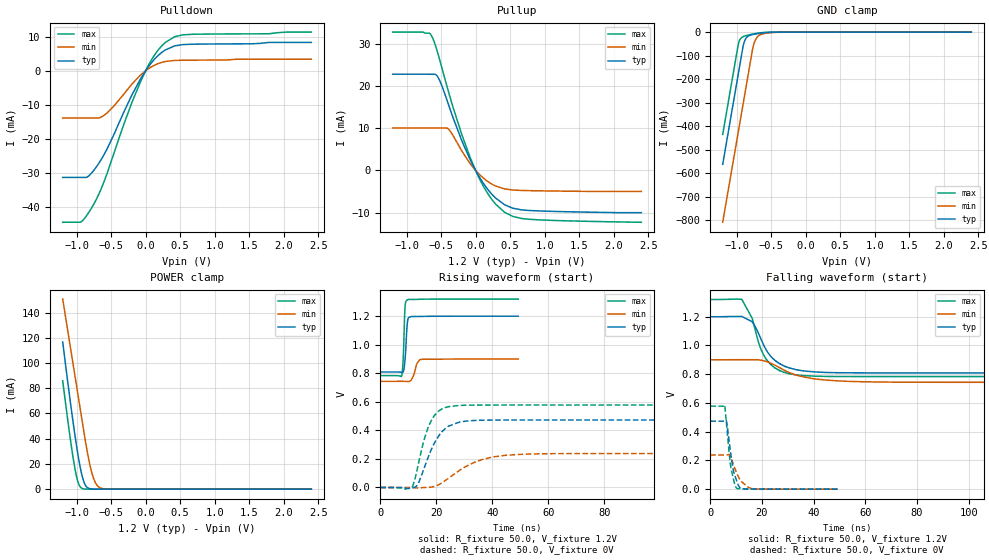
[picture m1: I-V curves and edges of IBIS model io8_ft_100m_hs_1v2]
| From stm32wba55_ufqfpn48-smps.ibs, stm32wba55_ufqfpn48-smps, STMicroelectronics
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[Model]   io8_ft_100m_hs_1v2
Model_type I/O
Polarity   Non-Inverting
Enable   Active-Low
| CAP_THRESHOLD on pad IOFT is "UDTCAPC" :
| Rising=30.0% of vddiom   Falling=70.0% of vddiom
| C_comp min and max val. don't necessarily correlate with the min and max pvt
| but are the smallest and greatest pad capacitance found.
| var   typ   min   max
C_comp   1.75103pF  1.57484pF  1.87847pF
|C_comp_pullup   1.05650pF  962.72500fF  1.08780pF
|C_comp_pulldown   694.52500fF  612.11500fF  790.67000fF
Vinl = 450.0mV
Vinh = 660.0mV
Vmeas = 600.0mV   | Reference voltage for timing measurements
Cref  = 50.0pF   | Timing specification test load capacitance value
Rref  = 1.0MOhm   | Timing specification test load resistance value
Vref  = 660.0mV   | Timing specification test load voltage
[Model Spec]
| TIME_THRESHOLD on pin ZIV11 is "CMOS" :
| Rising=50.0% of vdd   Falling=50.0% of vdd
Vinl 441.50000mV 347.50000mV 471.50000mV
Vinh 755.50000mV 552.50000mV 842.50000mV
| variable   typ   min   max
[Temperature Range] 25.0 140.0 -40.0
| variable   typ   min   max
[Voltage Range] 1.2V 900.0mV 1.32V
| variable   typ   min   max
[POWER Clamp Reference] 1.2V 900.0mV 1.32V
| variable   typ   min   max
[GND Clamp Reference] 0V 0V 0V
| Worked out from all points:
|   slope of the pulldown table from 0 to 0.18 V, typ, clamps not added: 40.6 ohm
|   slope of the pullup table from 0 to 0.18 V, typ, clamps not added: 39.4 ohm
|   GND clamp passes 1 mA (typ) near -0.51 V on its own axis
|   POWER clamp passes 1 mA (typ) near -0.83 V on its own axis
|   rising waveform, R_fixture 50.0, V_fixture 1.2V: 20-80 % time 738ps typ, 1.44ns min, 563ps max; typ from 0.809 V to 1.2 V
|   falling waveform, R_fixture 50.0, V_fixture 1.2V: 20-80 % time 8.08ns typ, 13.6ns min, 6.71ns max; typ from 1.2 V to 0.809 V
|   rising waveform, R_fixture 50.0, V_fixture 0V: 20-80 % time 6.62ns typ, 12.4ns min, 5ns max; typ from 0 V to 0.473 V
|   falling waveform, R_fixture 50.0, V_fixture 0V: 20-80 % time 2.5ns typ, 3.86ns min, 2.13ns max; typ from 0.473 V to 0 V
[POWER Clamp]
-1.2V     116.7mA    150.7mA    85.92mA
-1.06V    57.23mA    102.6mA    28.68mA
-1.02V    41.75mA    88.91mA    15.5mA
-980mV    27.6mA     75.18mA    5.935mA
-920mV    10.75mA    54.6mA     597.6uA
-870mV    3.065mA    37.68mA    60.82uA
-820mV    594.6uA    22.85mA    5.912uA
-770mV    99.71uA    11.47mA    572nA
-730mV    23.34uA    5.552mA    88.29nA
-680mV    3.779uA    1.833mA    8.565nA
-510mV    7.889nA    23.13uA    53.67pA
2.4V      0A         0A         0A
[GND Clamp]
-1.2V     -561.6mA   -807.5mA   -434.8mA
-980mV    -187.6mA   -433.5mA   -60.76mA
-960mV    -153.6mA   -399.5mA   -38.21mA
-900mV    -54.17mA   -297.5mA   -18.87mA
-870mV    -29.55mA   -246.5mA   -15.73mA
-830mV    -17.05mA   -178.5mA   -12.57mA
-760mV    -9.921mA   -62.77mA   -8.045mA
-730mV    -8.191mA   -35.56mA   -6.403mA
-680mV    -5.826mA   -15.57mA   -4.089mA
-580mV    -2.43mA    -5.043mA   -1.157mA
-330mV    -11.72uA   -245.5uA   -300.5nA
2.4V      872pA      1.056uA    338.3pA
| variable   typ   min   max
[Pullup Reference] 1.2V 900.0mV 1.32V
| variable   typ   min   max
[Pulldown Reference] 0V 0V 0V
[Pullup]
-1.2V     22.83mA    10.04mA    32.82mA
-760mV    22.83mA    10.04mA    32.82mA
-640mV    22.81mA    10.04mA    32.01mA
-580mV    22.78mA    10.04mA    29.58mA
-540mV    21.98mA    10.04mA    27.42mA
-390mV    15.52mA    9.757mA    18.55mA
-200mV    7.069mA    4.63mA     8.528mA
-30mV     926.7uA    571.2uA    1.132mA
190mV     -4.777mA   -2.782mA   -5.837mA
420mV     -8.158mA   -4.403mA   -9.943mA
790mV     -9.528mA   -4.812mA   -11.62mA
2.4V      -10.04mA   -4.994mA   -12.3mA
[Pulldown]
-1.2V     -31.2mA    -13.81mA   -44.3mA
-940mV    -31.2mA    -13.81mA   -44.26mA
-850mV    -31.11mA   -13.81mA   -42.26mA
-760mV    -29.39mA   -13.81mA   -39.38mA
-660mV    -26.52mA   -13.68mA   -35.32mA
-550mV    -22.55mA   -12.17mA   -29.6mA
-330mV    -12.74mA   -7.204mA   -16.5mA
-80mV     -2.622mA   -1.37mA    -3.49mA
110mV     2.963mA    1.428mA    3.999mA
290mV     6.144mA    2.737mA    8.347mA
540mV     7.674mA    3.096mA    10.53mA
2.4V      8.312mA    3.389mA    11.33mA
[Ramp]
dV/dt_r 283.79685mV/6.56055ns 142.77757mV/12.31742ns 346.62063mV/4.96214ns
dV/dt_f 234.65963mV/7.91256ns 93.76558mV/13.21647ns 321.77311mV/6.31648ns
R_load = 50.0
| Removed startup time: 0s 0s 0s  .
| Removed end time: 49.25ns.
[Rising Waveform]
R_fixture   = 50.0
V_fixture   = 1.2V
V_fixture_min = 900.0mV
V_fixture_max = 1.32V
0s        808.9mV    743.7mV    783.7mV
7.6ns     806.1mV    743.8mV    780.8mV
7.9ns     804.4mV    743.8mV    819.9mV
8.25ns    812.8mV    743.7mV    931.3mV
8.65ns    860mV      743.6mV    1.184V
8.85ns    900.3mV    743.5mV    1.267V
9.65ns    1.15V      742.6mV    1.314V
11.05ns   1.197V     751.7mV    1.317V
14.1ns    1.198V     895.5mV    1.319V
49.25ns   1.2V       900mV      1.32V
| Removed startup time: 0s 0s 0s  .
| Removed end time: 199.25ns.
[Falling Waveform]
R_fixture   = 50.0
V_fixture   = 1.2V
V_fixture_min = 900.0mV
V_fixture_max = 1.32V
0s        1.2V       900mV      1.32V
12.2ns    1.202V     900.8mV    1.321V
16.25ns   1.164V     900.8mV    1.188V
18.85ns   1.077V     899.4mV    1.011V
21.45ns   975.4mV    889.6mV    908.9mV
25.45ns   888.9mV    858.9mV    839.7mV
32.55ns   834.6mV    797.8mV    796.9mV
40.65ns   815.5mV    766.6mV    786.2mV
58.05ns   809.2mV    747.8mV    783.6mV
199.3ns   808.9mV    743.7mV    783.7mV
| Removed startup time: 0s 0s 0s  .
| Removed end time: 199.25ns.
[Rising Waveform]
R_fixture   = 50.0
V_fixture   = 0V
V_fixture_min = 0V
V_fixture_max = 0V
0s        4.648nV    985.5nV    3.924nV
11.45ns   -909.8uV   -1.529mV   6.784mV
13.6ns    30.33mV    -3.415mV   165.4mV
15.75ns   140.5mV    16.15uV    341.1mV
17.7ns    243mV      1.663mV    449.9mV
20.3ns    344.1mV    14.26mV    527mV
24.4ns    430mV      65.43mV    566.3mV
34.75ns   470.4mV    185.7mV    577.3mV
48.8ns    472.8mV    231.1mV    577.6mV
199.3ns   473mV      238mV      577.7mV
| Removed startup time: 0s 0s 0s  .
| Removed end time: 49.25ns.
[Falling Waveform]
R_fixture   = 50.0
V_fixture   = 0V
V_fixture_min = 0V
V_fixture_max = 0V
0s        473mV      238mV      577.7mV
5.55ns    472.6mV    238mV      584.6mV
6.3ns     469.4mV    237.8mV    451.6mV
7.3ns     332.8mV    241.5mV    252.4mV
7.95ns    242.6mV    220.6mV    152.2mV
9.05ns    121.7mV    165.8mV    63.97mV
10.3ns    53.56mV    108.8mV    5.172mV
11.8ns    4.87mV     58.64mV    1.947mV
16.1ns    1.011mV    4.188mV    718.7uV
49.25ns   1.919uV    31.21uV    -84.73nV
